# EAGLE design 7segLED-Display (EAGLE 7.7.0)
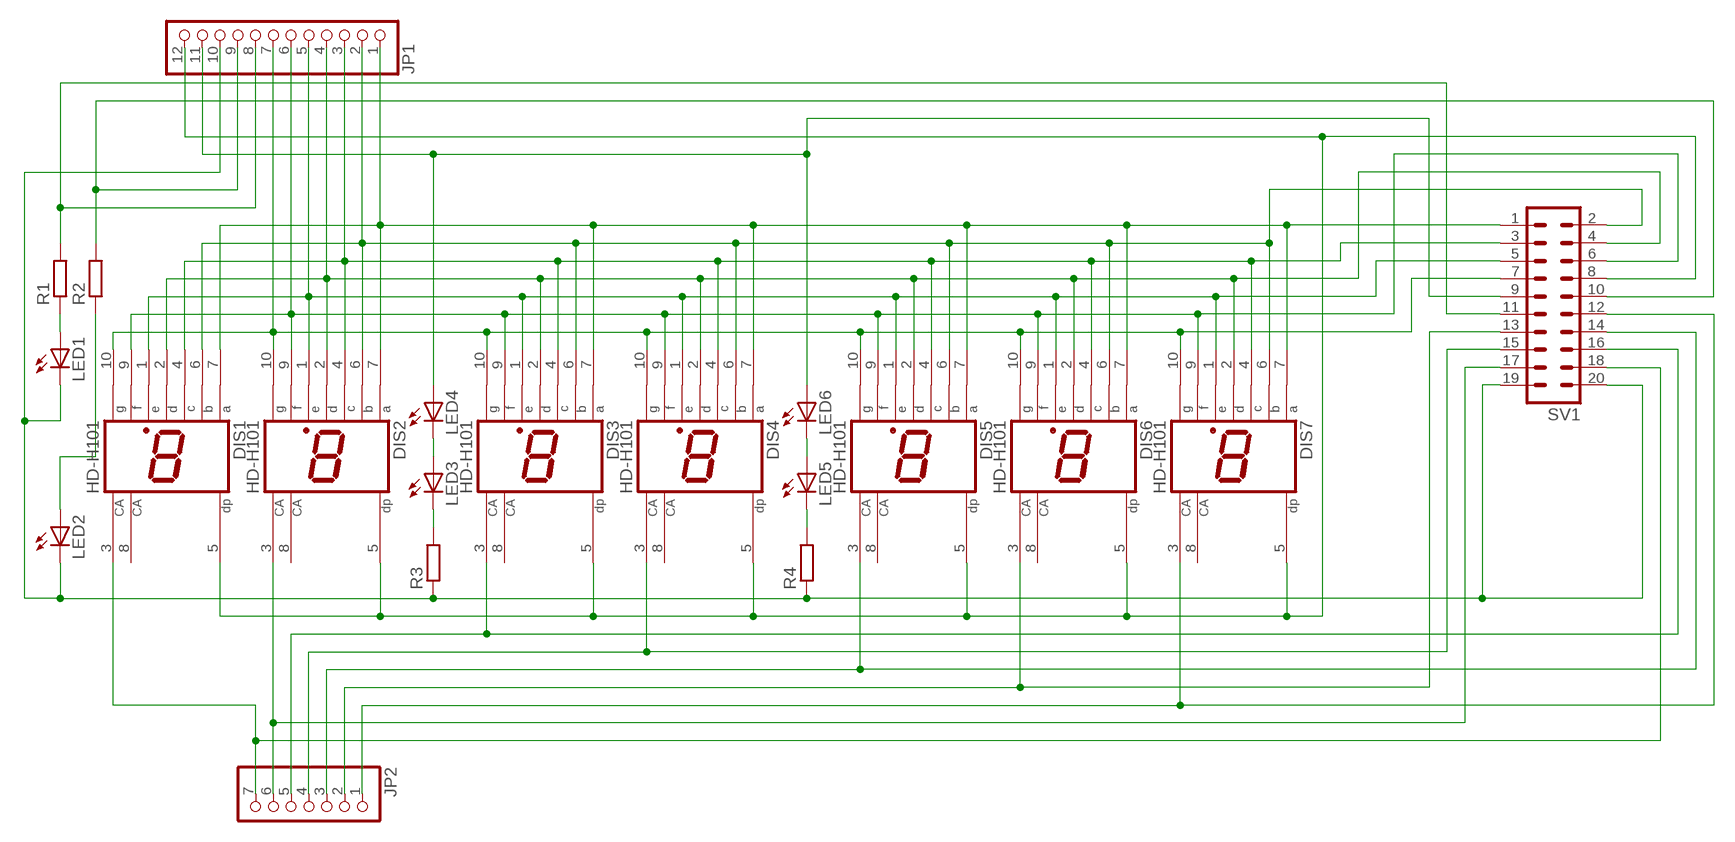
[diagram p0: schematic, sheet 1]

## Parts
DIS1  HD-H101  [HDSP-M]
DIS2  HD-H101  [HDSP-M]
DIS3  HD-H101  [HDSP-M]
DIS4  HD-H101  [HDSP-M]
DIS5  HD-H101  [HDSP-M]
DIS6  HD-H101  [HDSP-M]
DIS7  HD-H101  [HDSP-M]
JP1  PINHD-1X12  [1X12]
JP2  PINHD-1X7  [1X07]
LED1  LED5MM  [LED5MM]
LED2  LED5MM  [LED5MM]
LED3  LED3MM  [LED3MM]
LED4  LED3MM  [LED3MM]
LED5  LED3MM  [LED3MM]
LED6  LED3MM  [LED3MM]
R1  R-EU_M1206  [M1206]
R2  R-EU_M1206  [M1206]
R3  R-EU_M1206  [M1206]
R4  R-EU_M1206  [M1206]
SV1  ML20  [ML20]

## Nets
N$1: DIS1.9(F) DIS2.9(F) DIS3.9(F) DIS4.9(F) DIS5.9(F) DIS6.9(F) DIS7.9(F) JP1.6 SV1.6
N$2: DIS1.1(E) DIS2.1(E) DIS3.1(E) DIS4.1(E) DIS5.1(E) DIS6.1(E) DIS7.1(E) JP1.5 SV1.5
N$3: DIS1.2(D) DIS2.2(D) DIS3.2(D) DIS4.2(D) DIS5.2(D) DIS6.2(D) DIS7.2(D) JP1.4 SV1.4
N$4: DIS1.4(C) DIS2.4(C) DIS3.4(C) DIS4.4(C) DIS5.4(C) DIS6.4(C) DIS7.4(C) JP1.3 SV1.3
N$5: DIS1.6(B) DIS2.6(B) DIS3.6(B) DIS4.6(B) DIS5.6(B) DIS6.6(B) DIS7.6(B) JP1.2 SV1.2
N$6: DIS1.7(A) DIS2.7(A) DIS3.7(A) DIS4.7(A) DIS5.7(A) DIS6.7(A) DIS7.7(A) JP1.1 SV1.1
N$7: DIS1.10(G) DIS2.10(G) DIS3.10(G) DIS4.10(G) DIS5.10(G) DIS6.10(G) DIS7.10(G) JP1.7 SV1.7
N$8: JP1.8 R1.2 SV1.11
N$9: JP1.9 R2.2 SV1.10
N$10: JP1.10 LED1.K(C) LED2.K(C) R3.1 R4.1 SV1.19 SV1.20
N$11: DIS1.3(CA) JP2.7 SV1.18
N$12: DIS6.3(CA) JP2.2 SV1.13
N$13: DIS5.3(CA) JP2.3 SV1.14
N$14: DIS4.3(CA) JP2.4 SV1.15
N$15: DIS3.3(CA) JP2.5 SV1.16
N$16: DIS2.3(CA) JP2.6 SV1.17
N$17: LED3.A LED4.K(C)
N$18: LED3.K(C) R3.2
N$19: LED5.A LED6.K(C)
N$20: LED5.K(C) R4.2
N$21: JP1.11 LED4.A LED6.A SV1.9
N$39: DIS7.3(CA) JP2.1 SV1.12
N$40: DIS1.5(DP) DIS2.5(DP) DIS3.5(DP) DIS4.5(DP) DIS5.5(DP) DIS6.5(DP) DIS7.5(DP) JP1.12 SV1.8
N$41: LED2.A R2.1
N$42: LED1.A R1.1
Unconnected: DIS1.8(CA) DIS2.8(CA) DIS3.8(CA) DIS4.8(CA) DIS5.8(CA) DIS6.8(CA) DIS7.8(CA)

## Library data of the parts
DIS1-DIS7 = display-hp:HD-H101: LED DISPLAY 1-character 7 segment, decimal point right
JP1 = pinhead:PINHD-1X12: PIN HEADER
JP2 = pinhead:PINHD-1X7: PIN HEADER
LED1-LED6 = led:LED: LED
R1-R4 = rcl:R-EU_: RESISTOR, European symbol
SV1 = con-ml:ML20: HARTING; OC_FARNELL: unknown; OC_NEWARK: unknown

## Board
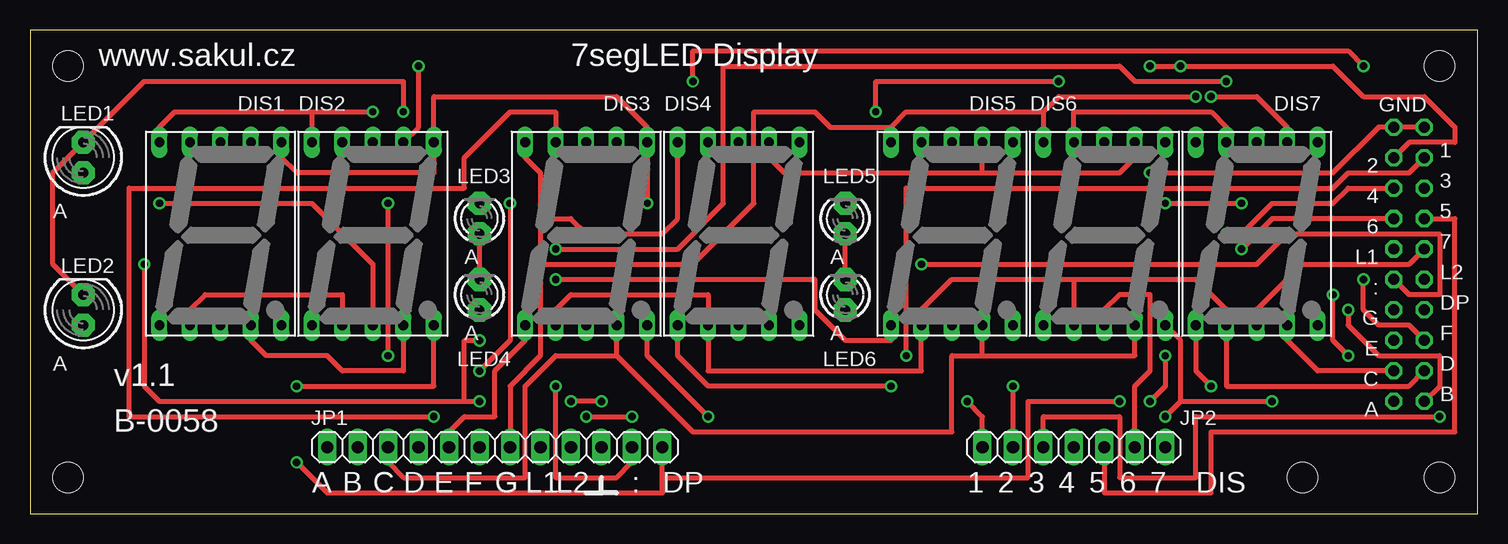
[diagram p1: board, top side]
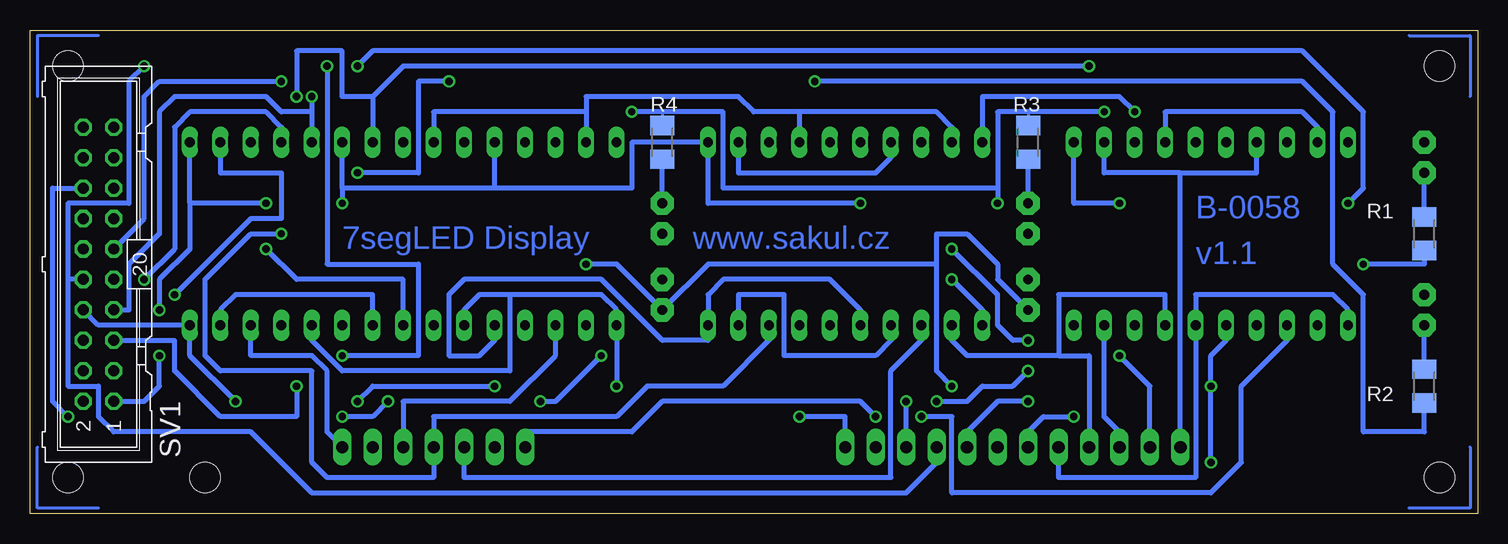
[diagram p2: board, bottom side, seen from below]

Size 120.63 x 40.31 mm. Coordinates in mm from the lower left corner, seen from the top.
Outline: 0,0 120.63,0 120.63,40.31 0,40.31 0,0
Copper layers (1*16): Top 0.035mm / dielectric 1.5mm / Bottom 0.035mm
Design rules "default": minimum track width 10mil, minimum drill 24mil, track to track 8mil, track to pad 8mil, pad to pad 8mil, via to via 8mil, smd to smd 8mil, copper to edge 40mil, drill to drill 8mil, minimum pad ring 10mil, minimum via ring 8mil, stop-mask expansion 4mil, vias tented up to drill 0mil, thermal gap 10mil
Holes 2.54 mm at 3.17,37.3 3.17,3.01 117.47,37.3 117.47,3.01 106.04,3.01

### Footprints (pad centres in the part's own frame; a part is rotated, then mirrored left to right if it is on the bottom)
HDSP-M = drill 0.813 long: 1 -5.08,-7.62; 2 -2.54,-7.62; 3 0,-7.62; 4 2.54,-7.62; 5 5.08,-7.62; 6 5.08,7.62; 7 2.54,7.62; 8 0,7.62; 9 -2.54,7.62; 10 -5.08,7.62
1X12 = drill 1.016 long: 1 -13.97,0; 2 -11.43,0; 3 -8.89,0; 4 -6.35,0; 5 -3.81,0; 6 -1.27,0; 7 1.27,0; 8 3.81,0; 9 6.35,0; 10 8.89,0; 11 11.43,0; 12 13.97,0
1X07 = drill 1.016 long: 1 -7.62,0; 2 -5.08,0; 3 -2.54,0; 4 0,0; 5 2.54,0; 6 5.08,0; 7 7.62,0
LED5MM = drill 0.813 pad 1.93 octagon: A -1.27,0; K 1.27,0
LED3MM = drill 0.813 pad 1.93 octagon: A -1.27,0; K 1.27,0
M1206 = smd 1.6 x 2: 1 -1.4,0; 2 1.4,0
ML20 = drill 0.914 octagon: 1 -11.43,-1.27; 2 -11.43,1.27; 3 -8.89,-1.27; 4 -8.89,1.27; 5 -6.35,-1.27; 6 -6.35,1.27; 7 -3.81,-1.27; 8 -3.81,1.27; 9 -1.27,-1.27; 10 -1.27,1.27; 11 1.27,-1.27; 12 1.27,1.27; 13 3.81,-1.27; 14 3.81,1.27; 15 6.35,-1.27; 16 6.35,1.27; 17 8.89,-1.27; 18 8.89,1.27; 19 11.43,-1.27; 20 11.43,1.27

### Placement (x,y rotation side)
DIS1  15.87,23.33 0 top
DIS2  28.57,23.33 0 top
DIS3  46.35,23.33 0 top
DIS4  59.05,23.33 0 top
DIS5  76.83,23.33 0 top
DIS6  89.53,23.33 0 top
DIS7  102.23,23.33 0 top
JP1  38.73,5.55 0 top
JP2  86.99,5.55 180 top
LED1  4.44,29.68 90 top
LED2  4.44,16.98 90 top
LED3  37.46,24.6 90 top
LED4  37.46,18.25 90 top
LED5  67.94,24.6 90 top
LED6  67.94,18.25 90 top
R1  4.44,23.33 270 bottom
R2  4.44,10.63 270 bottom
R3  37.46,30.95 270 bottom
R4  67.94,30.95 270 bottom
SV1  114.93,20.79 90 bottom

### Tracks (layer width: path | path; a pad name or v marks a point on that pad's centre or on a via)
N$1  (via drill 0.61)
  Top 0.406: v33.65,8.09 8.25,8.09 8.25,27.14 13.33,27.14 | DIS7.9 99.69,32.22 98.42,33.49 86.99,33.49 DIS6.9 | 13.33,27.14 36.19,27.14 36.19,29.68 40,33.49 43.81,33.49 DIS3.9 | 13.33,27.14 DIS1.9 | v111.12,19.52 111.12,16.98 112.39,15.71 114.93,15.71 SV1.6
  Bottom 0.406: DIS1.9 13.33,32.22 14.6,33.49 26.03,33.49 DIS2.9 | v33.65,8.09 36.19,8.09 37.46,6.82 JP1.6 | 56.51,33.49 45.08,33.49 43.81,32.22 DIS3.9 | 56.51,33.49 DIS4.9 | 74.29,33.49 86.99,33.49 DIS6.9 | 74.29,33.49 DIS5.9 | v111.12,19.52 108.58,22.06 108.58,32.22 107.31,33.49 100.96,33.49 99.69,32.22 DIS7.9 | 56.51,33.49 60.32,33.49 61.59,34.76 74.29,34.76 74.29,33.49
N$2  (via drill 0.61)
  Top 0.406: DIS3.1 41.27,14.44 38.73,11.9 38.73,8.09 36.19,8.09 34.92,6.82 JP1.5 | v71.75,10.63 56.51,10.63 53.97,13.17 DIS4.1 | v98.42,10.63 97.15,11.9 DIS7.1 | v43.81,19.52 65.4,19.52 65.4,16.98 67.94,14.44 71.75,14.44 DIS5.1
  Bottom 0.406: DIS1.1 10.79,16.98 12.06,18.25 23.49,18.25 DIS2.1 23.49,3.01 34.92,3.01 JP1.5 | v71.75,10.63 DIS5.1 71.75,16.98 73.02,18.25 80.64,18.25 | 80.64,18.25 83.18,18.25 84.45,16.98 DIS6.1 | 80.64,18.25 80.64,11.9 94.61,11.9 97.15,14.44 DIS7.1 | v98.42,10.63 98.42,8.09 104.77,8.09 108.58,11.9 108.58,14.44 SV1.5 | v43.81,19.52 41.27,16.98 DIS3.1
N$3
  Top 0.254: 99.69,16.98 DIS7.2
  Top 0.406: 86.99,19.52 76.83,19.52 74.29,16.98 DIS5.2 74.29,11.9 56.51,11.9 DIS4.2 56.51,18.25 45.08,18.25 43.81,16.98 DIS3.2 | 86.99,19.52 DIS6.2 | 99.69,16.98 97.15,19.52 86.99,19.52 | DIS7.2 99.69,10.63 114.93,10.63 SV1.4 | DIS1.2 13.33,16.98 14.6,18.25 26.03,18.25 DIS2.2
  Bottom 0.406: 34.92,13.17 32.38,13.17 JP1.4 | 34.92,13.17 34.92,18.25 26.03,18.25 DIS2.2 | 34.92,13.17 42.54,13.17 43.81,14.44 DIS3.2
N$4
  Top 0.406: DIS1.4 18.41,14.44 19.68,13.17 24.76,13.17 26.03,11.9 31.11,11.9 DIS2.4 | DIS7.4 104.77,14.44 107.31,11.9 SV1.3 | 79.37,13.17 92.07,13.17 DIS6.4 | 79.37,13.17 DIS5.4 | 48.89,13.17 55.24,6.82 76.83,6.82 76.83,13.17 79.37,13.17 | 48.89,13.17 43.81,13.17 41.27,10.63 41.27,3.01 31.11,3.01 29.84,4.28 JP1.3 | 48.89,13.17 DIS3.4
  Bottom 0.406: JP1.3 29.84,6.82 31.11,8.09 DIS2.4 | DIS3.4 48.89,14.44 50.16,13.17 57.78,13.17 57.78,18.25 61.59,18.25 DIS4.4 | DIS7.4 104.77,16.98 103.5,18.25 92.07,18.25 DIS6.4
N$5  (via drill 0.61)
  Top 0.406: DIS1.6 20.95,29.68 22.22,28.41 33.65,28.41 DIS2.6 33.65,34.76 48.89,34.76 51.43,32.22 DIS3.6 v51.43,25.87 | v29.84,13.17 v29.84,25.87 | v109.85,16.98 109.85,15.71 112.39,13.17 117.47,13.17 117.47,10.63 SV1.2 | v94.61,25.87 v100.96,25.87
  Bottom 0.406: v29.84,13.17 27.3,10.63 JP1.2 | v29.84,25.87 33.65,25.87 DIS2.6 | 107.31,25.87 107.31,22.06 109.85,19.52 v109.85,16.98 | 107.31,25.87 DIS7.6 | 81.91,27.14 70.48,27.14 70.48,30.95 DIS4.6 64.13,25.87 v51.43,25.87 | 81.91,27.14 DIS5.6 | 81.91,27.14 94.61,27.14 | 94.61,27.14 DIS6.6 | v100.96,25.87 107.31,25.87 | 94.61,27.14 v94.61,25.87
N$6  (via drill 0.61)
  Top 0.254: 104.77,32.22 DIS7.7
  Top 0.406: 104.77,32.22 102.23,34.76 v98.42,34.76 | v109.85,13.17 108.58,14.44 v108.58,18.25 | 79.37,28.41 62.86,28.41 61.59,29.68 DIS4.7 | 79.37,28.41 DIS5.7 | DIS2.7 32.38,32.22 v32.38,37.3 | 79.37,28.41 90.8,28.41 92.07,29.68 DIS6.7
  Bottom 0.406: 24.76,28.41 18.41,28.41 DIS1.7 | JP1.1 24.76,28.41 | 24.76,28.41 31.11,28.41 DIS2.7 | DIS3.7 48.89,29.68 50.16,28.41 61.59,28.41 DIS4.7 | v98.42,34.76 98.42,38.57 94.61,38.57 94.61,34.76 92.07,34.76 | v108.58,18.25 102.23,24.6 99.69,24.6 99.69,28.41 104.77,28.41 DIS7.7 | v32.38,37.3 89.53,37.3 92.07,34.76 | 92.07,34.76 DIS6.7 | SV1.1 111.12,9.36 109.85,10.63 v109.85,13.17
N$7  (via drill 0.61)
  Top 0.406: 71.75,32.22 73.02,33.49 84.45,33.49 | 84.45,33.49 DIS6.10 | v97.15,34.76 85.72,34.76 84.45,33.49 | 23.49,33.49 12.06,33.49 10.79,32.22 DIS1.10 | 23.49,33.49 DIS2.10 | DIS3.10 41.27,29.68 42.54,28.41 42.54,24.6 | 42.54,24.6 42.54,20.79 | 42.54,20.79 42.54,13.17 40,10.63 JP1.7 | 23.49,33.49 v28.57,33.49 | 71.75,32.22 66.67,32.22 65.4,33.49 60.32,33.49 60.32,25.87 55.24,20.79 42.54,20.79 | 71.75,32.22 DIS5.10 | DIS4.10 53.97,24.6 52.7,23.33 46.35,23.33 45.08,24.6 42.54,24.6
  Bottom 0.406: 97.15,33.49 DIS7.10 | v97.15,34.76 97.15,33.49 | v28.57,33.49 29.84,34.76 41.27,34.76 DIS3.10 | 97.15,33.49 99.69,33.49 100.96,34.76 108.58,34.76 109.85,33.49 109.85,23.33 112.39,20.79 112.39,16.98 SV1.7
N$8  (via drill 0.61)
  Top 0.406: v9.52,20.79 9.52,10.63 10.79,9.36 36.19,9.36 | 36.19,9.36 v37.46,9.36 | v99.69,36.03 92.07,36.03 90.8,37.3 57.78,37.3 57.78,25.87 53.97,22.06 v43.81,22.06 | v37.46,14.44 36.19,14.44 36.19,9.36
  Bottom 0.254: R1.2 4.44,22.06
  Bottom 0.406: v37.46,9.36 40,9.36 42.54,6.82 JP1.8 | v99.69,36.03 109.85,36.03 111.12,34.76 111.12,24.6 SV1.11 | v43.81,22.06 40,18.25 40,15.71 38.73,14.44 v37.46,14.44 | v9.52,20.79 4.44,20.79 4.44,22.06
N$9  (via drill 0.61)
  Top 0.406: v55.24,36.03 55.24,38.57 109.85,38.57 v111.12,37.3
  Bottom 0.406: v55.24,36.03 14.6,36.03 12.06,33.49 12.06,20.79 9.52,18.25 9.52,6.82 4.44,6.82 R2.2 | v111.12,37.3 112.39,36.03 112.39,25.87 117.47,25.87 117.47,19.52 | 117.47,19.52 117.47,10.63 114.93,10.63 114.93,8.09 113.66,6.82 102.23,6.82 97.15,1.74 47.62,1.74 45.08,4.28 JP1.9 | SV1.10 117.47,19.52
N$10  (via drill 0.61)
  Top 0.406: LED2.K 1.9,20.79 1.9,28.41 LED1.K 9.52,36.03 31.11,36.03 v31.11,33.49 | v47.62,9.36 v45.08,9.36 | v37.46,11.9 40,14.44 v40,25.87 | v93.34,28.41 108.58,28.41 112.39,32.22 SV1.19 SV1.20 | v85.72,36.03 70.48,36.03 v70.48,33.49
  Bottom 0.254: 67.94,33.49 R4.1 67.94,32.22 | 37.46,33.49 R3.1
  Bottom 0.406: 40,27.14 40,33.49 37.46,33.49 v31.11,33.49 | 40,27.14 62.86,27.14 62.86,33.49 67.94,33.49 v70.48,33.49 | v37.46,11.9 38.73,10.63 41.27,10.63 42.54,9.36 v45.08,9.36 | 40,27.14 v40,25.87 | JP1.10 v47.62,9.36 | v93.34,28.41 88.26,28.41 88.26,36.03 v85.72,36.03
N$11  (via drill 0.61)
  Top 0.406: v46.35,8.09 v50.16,8.09 | v73.02,13.17 73.02,27.14 108.58,27.14 109.85,28.41 114.93,28.41 SV1.18 | v78.1,9.36 79.37,8.09 JP2.7
  Bottom 0.406: v46.35,8.09 43.81,8.09 43.81,1.74 22.22,1.74 19.68,4.28 19.68,10.63 15.87,14.44 DIS1.3 | v50.16,8.09 51.43,9.36 67.94,9.36 70.48,6.82 79.37,6.82 JP2.7 | v73.02,13.17 76.83,9.36 v78.1,9.36
N$12  (via drill 0.61)
  Top 0.406: DIS6.3 89.53,16.98 90.8,18.25 93.34,18.25 93.34,11.9 92.07,10.63 JP2.2 | v100.96,22.06 103.5,24.6 SV1.13
  Bottom 0.406: v100.96,22.06 98.42,19.52 89.53,19.52 DIS6.3
N$13
  Top 0.406: JP2.3 89.53,1.74 98.42,1.74 98.42,6.82 118.74,6.82 118.74,24.6 SV1.14
  Bottom 0.406: DIS5.3 76.83,13.17 80.64,9.36 89.53,9.36 JP2.3
N$14  (via drill 0.61)
  Top 0.406: v99.69,23.33 100.96,23.33 103.5,25.87 108.58,25.87 109.85,27.14 SV1.15
  Bottom 0.406: DIS4.3 59.05,14.44 62.86,10.63 69.21,10.63 71.75,8.09 86.99,8.09 JP2.4 86.99,3.01 95.88,3.01 97.15,4.28 97.15,11.9 104.77,11.9 106.04,13.17 106.04,19.52 102.23,23.33 v99.69,23.33
N$15  (via drill 0.61)
  Top 0.406: v117.47,8.09 97.15,8.09 97.15,3.01 90.8,3.01 90.8,8.09 84.45,8.09 JP2.5
  Bottom 0.406: DIS3.3 46.35,14.44 48.89,11.9 48.89,3.01 84.45,3.01 JP2.5 | v117.47,8.09 118.74,9.36 118.74,27.14 SV1.16
N$16  (via drill 0.61)
  Top 0.406: v10.79,25.87 23.49,25.87 28.57,20.79 DIS2.3 | v93.34,37.3 v95.88,37.3 108.58,37.3 111.12,34.76 116.2,34.76 118.74,32.22 118.74,30.95 114.93,30.95 SV1.17 | v93.34,9.36 94.61,10.63 v94.61,13.17 | v81.91,10.63 JP2.6
  Bottom 0.406: v10.79,25.87 9.52,27.14 9.52,33.49 14.6,38.57 92.07,38.57 v93.34,37.3 | v81.91,10.63 92.07,10.63 v93.34,9.36 | v94.61,13.17 88.26,13.17 88.26,20.79 95.88,20.79 v95.88,37.3
N$17
  Top 0.406: LED4.K LED3.A
N$18
  Bottom 0.254: R3.2 37.46,29.68
  Bottom 0.406: LED3.K R3.2
N$19
  Top 0.406: LED6.K LED5.A
N$20
  Bottom 0.254: R4.2 67.94,29.68
  Bottom 0.406: LED5.K R4.2
N$21  (via drill 0.61)
  Top 0.406: v43.81,10.63 43.81,3.01 48.89,3.01 50.16,4.28 JP1.11 | v74.29,20.79 102.23,20.79 104.77,23.33 117.47,23.33 117.47,18.25 114.93,18.25 SV1.9
  Bottom 0.406: v43.81,10.63 45.08,11.9 45.08,20.79 | 45.08,20.79 64.13,20.79 LED6.A 71.75,20.79 v74.29,20.79 | 45.08,20.79 45.08,23.33 42.54,23.33 40,20.79 40,19.52 LED4.A
N$22
  Bottom 0.254: 5.71,39.84 0.63,39.84 0.63,34.76
N$23
  Bottom 0.254: 0.63,5.55 0.63,0.47 5.71,0.47
N$24
  Bottom 0.254: 114.93,0.47 120.01,0.47 120.01,5.55
N$25
  Bottom 0.254: 114.93,39.84 120.01,39.84 120.01,34.76
N$39
  Top 0.406: DIS7.3 102.23,16.98 106.04,20.79 114.93,20.79 SV1.12
  Bottom 0.406: JP2.1 95.88,6.82 95.88,11.9 97.15,13.17 102.23,13.17 DIS7.3
N$40  (via drill 0.61)
  Top 0.406: 95.88,9.36 95.88,14.44 DIS6.5 | 95.88,9.36 v103.5,9.36 | v22.22,10.63 33.65,10.63 DIS2.5 | v56.51,8.09 51.43,13.17 DIS3.5 | v22.22,4.28 24.76,1.74 52.7,1.74 52.7,3.01 | 52.7,3.01 JP1.12 | v94.61,8.09 95.88,9.36 | v90.8,9.36 83.18,9.36 83.18,3.01 52.7,3.01
  Bottom 0.254: 81.91,14.44 DIS5.5
  Bottom 0.406: v103.5,9.36 107.31,13.17 DIS7.5 114.93,15.71 SV1.8 | DIS1.5 20.95,14.44 22.22,13.17 v22.22,10.63 v22.22,4.28 | DIS3.5 51.43,16.98 53.97,19.52 62.86,19.52 64.13,18.25 DIS4.5 64.13,14.44 67.94,14.44 73.02,19.52 84.45,19.52 85.72,18.25 85.72,13.17 83.18,13.17 81.91,14.44 | v56.51,8.09 52.7,8.09 JP1.12 | v94.61,8.09 92.07,8.09 v90.8,9.36
N$41
  Bottom 0.254: R2.1 4.44,11.9
  Bottom 0.406: R2.1 LED2.A
N$42
  Bottom 0.254: R1.1 4.44,24.6
  Bottom 0.406: R1.1 LED1.A

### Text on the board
Bottom: B-0058 | www.sakul.cz | 7segLED Display | v1.1
tNames: www.sakul.cz | 7segLED Display | GND | 2 | 1 | 4 | 3 | A | 6 | 5 | L1 | 7 | A | A | : | L2 | G | DP | A | A | E | F | A | C | D | v1.1 | A | B | B-0058 | A | B | C | D | E | F | G | L1 | L2 | : | DP | 1 | 2 | 3 | 4 | 5 | 6 | 7 | DIS
bDocu: B-0004 | 7segLED Display | v1.0 | www.sakul.cz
